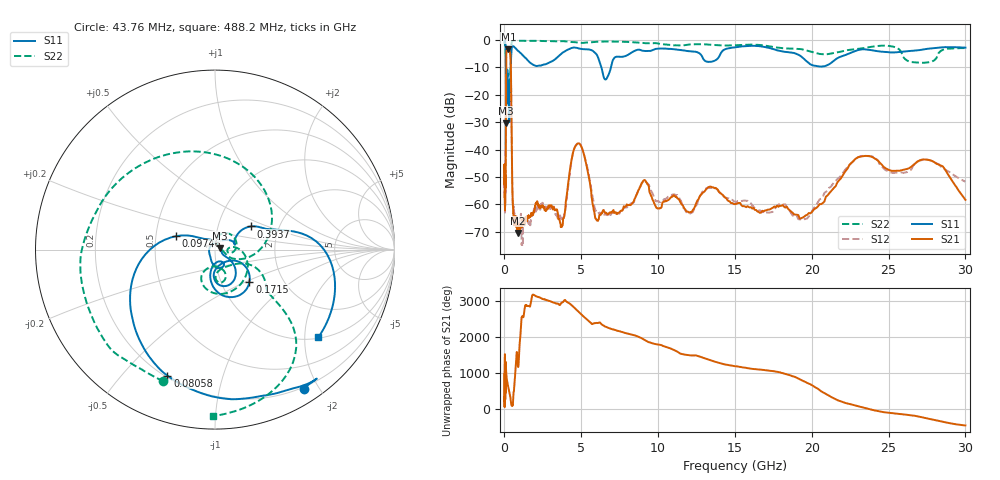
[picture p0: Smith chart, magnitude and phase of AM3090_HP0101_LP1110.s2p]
! Date/Time: Thu, Feb 28, 2019 1:59 PM
! Network Analyzer: Agilent Technologies E8364B Rev: A.07.50.67
! Sweep from 0.010 to 30.000 GHz, 1601 Points, Sweep Type: LOG
! Power Supply: 5.023 V, 0.002 A
# Hz S DB R 50
!freq MagS11 AngS11 MagS21 AngS21 MagS12 AngS12 MagS22 AngS22
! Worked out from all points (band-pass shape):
!   1601 points, 10 MHz to 30 GHz, reference 50 ohm
!   highest |S21| = -3.47 dB at 253.4 MHz (marker M1); lowest = -70.5 dB at 898.9 MHz (marker M2)
!   |S21| within 3 dB of the highest: 109.6 MHz to 396.8 MHz (287.1 MHz wide, 113 % of centre)
!   lowest |S11| = -30.5 dB at 105.6 MHz (marker M3), VSWR 1.06, Z = 53 + j0.88 ohm
!   |S11| at or under -10 dB: 95.93 MHz to 409.9 MHz (313.9 MHz wide, 124 % of centre); 6.308 GHz to 6.931 GHz (622.4 MHz wide, 9.4 % of centre)
!   |S22| runs from -31.1 to -0.2 dB; largest |S21 - S12| = 0.0095
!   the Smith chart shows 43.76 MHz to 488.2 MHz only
!   S11 on the Smith chart (normalised r, x): 43.76 MHz: 0.18, -1.81; 80.58 MHz: 0.21, -0.67; 97.46 MHz: 0.64, +0.10; 171.5 MHz: 1.36, -0.52; 393.7 MHz: 1.43, +0.39; 488.2 MHz: 1.03, -2.34
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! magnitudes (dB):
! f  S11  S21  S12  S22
! 10 MHz  -0.3  -45.7  -47.7  -0.7
! 38.04 MHz  -0.5  -59.2  -60.8  -1.6
! 43.76 MHz  -0.7  -58.0  -59.7  -2.1
! 80.58 MHz  -2.5  -48.9  -48.3  -4.6
! 97.46 MHz  -12.8  -15.3  -15.2  -13.2
! 105.6 MHz  -30.5  -7.7  -7.7  -30.9
! 120.2 MHz  -13.7  -5.1  -5.1  -18.5
! 144.7 MHz  -21.2  -3.9  -3.8  -23.3
! 171.5 MHz  -11.6  -3.6  -3.6  -14.3
! 253.4 MHz  -22.5  -3.5  -3.4  -17.7
! 393.7 MHz  -12.5  -6.2  -6.2  -10.3
! 488.2 MHz  -2.4  -44.8  -44.7  -0.7
! 550.5 MHz  -2.3  -60.6  -60.5  -0.4
! 898.9 MHz  -4.0  -70.5  -68.2  -0.3
! 2.084 GHz  -9.5  -59.9  -62.1  -0.3
! 3.742 GHz  -4.8  -68.2  -66.0  -0.4
! 4.781 GHz  -3.0  -37.8  -37.7  -1.0
! 5.989 GHz  -5.2  -65.6  -62.8  -0.7
! 7.926 GHz  -5.8  -60.6  -61.0  -0.7
! 19.31 GHz  -6.0  -65.0  -65.4  -3.4
! 23.48 GHz  -3.5  -42.3  -42.3  -2.9
! 30 GHz  -2.8  -58.3  -51.8  -3.0
